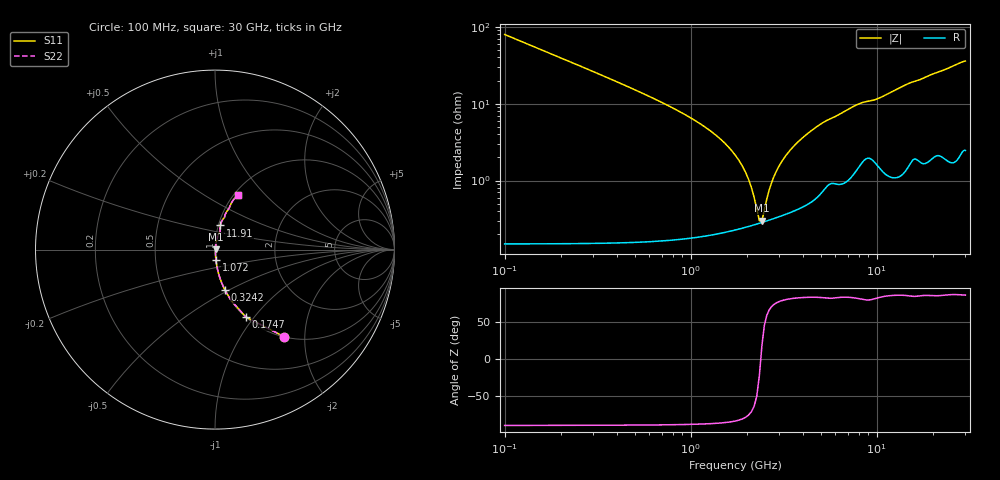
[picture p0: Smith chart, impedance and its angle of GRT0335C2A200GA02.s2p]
!Murata Part Number: GRT0335C2A200GA02
!These Parameters are Measured in Series Mode Connection
!Data Generated on Jun 19, 2026
!  o--ll--o
!Port1  Port2
!  o------o
!Operation Temp=25[degC], DC Bias Voltage=0[V]
!Freq. Start=100[MHz] Stop=30[GHz] 401[Steps]
# Hz S RI R 50
!Freq.(Hz) S11(Real) S11(Imag) S21(Real) S21(Imag) S12(Real) S12(Imag) S22(Real) S22(Imag)
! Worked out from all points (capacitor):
!   401 points, 100 MHz to 30 GHz, reference 50 ohm
!   read as one part in series: C = 20 pF near 249.5 MHz
!   lowest |Z| = 300 mohm at 2.417 GHz (marker M1)
!   series resonance near 2.383 GHz, so ESL is about 220 pH
!   S11 on the Smith chart (normalised r, x): 100 MHz: 1.00, -1.59; 174.8 MHz: 1.00, -0.91; 324.2 MHz: 1.00, -0.48; 1.072 GHz: 1.00, -0.12; 11.91 GHz: 1.02, +0.28; 30 GHz: 1.05, +0.72
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1e8  0.3871 -0.4861  0.6129 0.4861  0.6129 0.4861  0.3871 -0.4861
1.7475e8  0.171 -0.3749  0.829 0.3749  0.829 0.3749  0.171 -0.3749
3.2425e8  0.0561 -0.227  0.9439 0.227  0.9439 0.227  0.0561 -0.227
6.2325e8  0.0155 -0.1168  0.9845 0.1168  0.9845 0.1168  0.0155 -0.1168
1.07175e9  0.00527 -0.0586  0.9947 0.0586  0.9947 0.0586  0.00527 -0.0586
1.81925e9  0.00266 -0.018  0.9973 0.018  0.9973 0.018  0.00266 -0.018
2.0435e9  0.00262 -0.0102  0.9974 0.0102  0.9974 0.0102  0.00262 -0.0102
2.26775e9  0.00272 -0.00326  0.9973 0.00326  0.9973 0.00326  0.00272 -0.00326
2.41725e9  0.00284 0.000939  0.9972 -0.000939  0.9972 -0.000939  0.00284 0.000939
2.492e9  0.00292 0.00294  0.9971 -0.00294  0.9971 -0.00294  0.00292 0.00294
2.71625e9  0.00319 0.00862  0.9968 -0.00862  0.9968 -0.00862  0.00319 0.00862
2.86575e9  0.0034 0.0122  0.9966 -0.0122  0.9966 -0.0122  0.0034 0.0122
3.2395e9  0.00404 0.0204  0.996 -0.0204  0.996 -0.0204  0.00404 0.0204
3.987e9  0.00572 0.0352  0.9943 -0.0352  0.9943 -0.0352  0.00572 0.0352
5.10825e9  0.0101 0.0547  0.9899 -0.0547  0.9899 -0.0547  0.0101 0.0547
7.7245e9  0.0215 0.0912  0.9785 -0.0912  0.9785 -0.0912  0.0215 0.0912
1.01165e10  0.0277 0.1099  0.9723 -0.1099  0.9723 -0.1099  0.0277 0.1099
1.19105e10  0.0295 0.1343  0.9705 -0.1343  0.9705 -0.1343  0.0295 0.1343
1.505e10  0.0474 0.1732  0.9526 -0.1732  0.9526 -0.1732  0.0474 0.1732
2.005825e10  0.0717 0.2208  0.9283 -0.2208  0.9283 -0.2208  0.0717 0.2208
2.50665e10  0.0953 0.2665  0.9047 -0.2665  0.9047 -0.2665  0.0953 0.2665
3e10  0.1304 0.3042  0.8696 -0.3042  0.8696 -0.3042  0.1304 0.3042
